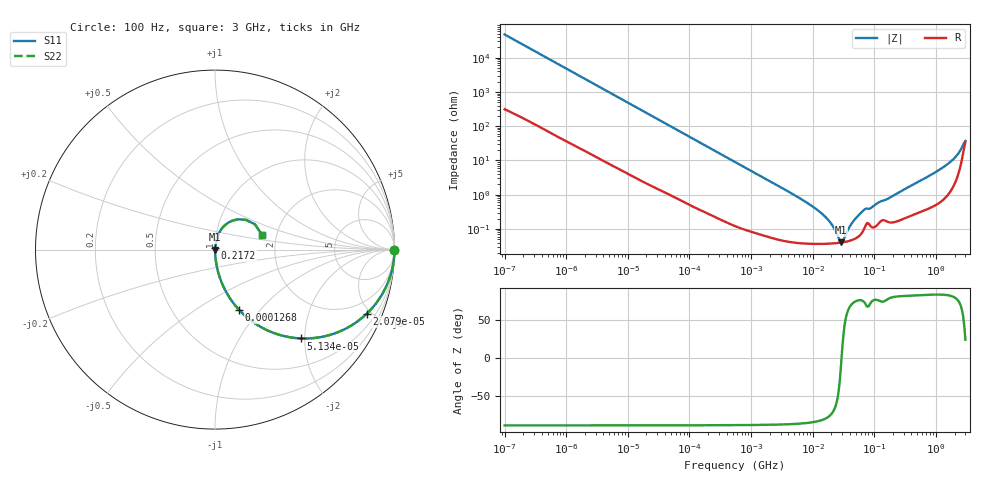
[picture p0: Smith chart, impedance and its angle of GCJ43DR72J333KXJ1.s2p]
!Murata Part Number: GCJ43DR72J333KXJ1
!These Parameters are Measured in Series Mode Connection
!Data Generated on Mar 13, 2026
!  o--ll--o
!Port1  Port2
!  o------o
!Operation Temp=25[degC], DC Bias Voltage=0[V]
!Freq. Start=100[Hz] Stop=3[GHz] 401[Steps]
# Hz S RI R 50
!Freq.(Hz) S11(Real) S11(Imag) S21(Real) S21(Imag) S12(Real) S12(Imag) S22(Real) S22(Imag)
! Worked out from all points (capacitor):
!   401 points, 100 Hz to 3 GHz, reference 50 ohm
!   read as one part in series: C = 33.4 nF near 109 Hz
!   lowest |Z| = 40.6 mohm at 28.73 MHz (marker M1)
!   series resonance near 29.37 MHz, so ESL is about 880 pH
!   S11 on the Smith chart (normalised r, x): 100 Hz: open; 20.79 kHz: 1.04, -4.70; 51.34 kHz: 1.02, -1.92; 126.8 kHz: 1.01, -0.78; 217.2 MHz: 1.00, +0.02; 3 GHz: 1.68, +0.30
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100  1 -0.0021  1.82e-05 0.0021  1.82e-05 0.0021  1 -0.0021
1788  0.9983 -0.0369  0.00166 0.0369  0.00166 0.0369  0.9983 -0.0369
6790  0.9798 -0.1367  0.0202 0.1367  0.0202 0.1367  0.9798 -0.1367
20793  0.8448 -0.3578  0.1552 0.3578  0.1552 0.3578  0.8448 -0.3578
31977  0.6999 -0.4538  0.3001 0.4538  0.3001 0.4538  0.6999 -0.4538
51340  0.4786 -0.4947  0.5214 0.4947  0.5214 0.4947  0.4786 -0.4947
126767  0.1346 -0.3361  0.8654 0.3361  0.8654 0.3361  0.1346 -0.3361
231582  0.046 -0.2039  0.954 0.2039  0.954 0.2039  0.046 -0.2039
547723  0.0094 -0.0901  0.9906 0.0901  0.9906 0.0901  0.0094 -0.0901
9794414  0.000387 -0.00459  0.9996 0.00459  0.9996 0.00459  0.000387 -0.00459
1.789277e7  0.000373 -0.00178  0.9996 0.00178  0.9996 0.00178  0.000373 -0.00178
2.12544e7  0.000378 -0.00114  0.9996 0.00114  0.9996 0.00114  0.000378 -0.00114
2.872754e7  0.000399 -7.66e-05  0.9996 7.66e-05  0.9996 7.66e-05  0.000399 -7.66e-05
3.131008e7  0.000409 0.000223  0.9996 -0.000223  0.9996 -0.000223  0.000409 0.000223
4.418008e7  0.000482 0.00148  0.9995 -0.00148  0.9995 -0.00148  0.000482 0.00148
6.508213e7  0.000858 0.00323  0.9991 -0.00323  0.9991 -0.00323  0.000858 0.00323
1.751444e8  0.00161 0.0079  0.9984 -0.0079  0.9984 -0.0079  0.00161 0.0079
2.172002e8  0.00169 0.00999  0.9983 -0.00999  0.9983 -0.00999  0.00169 0.00999
1.382454e9  0.0121 0.0659  0.9879 -0.0659  0.9879 -0.0659  0.0121 0.0659
2.219584e9  0.0496 0.1306  0.9504 -0.1306  0.9504 -0.1306  0.0496 0.1306
2.636591e9  0.1291 0.1688  0.8709 -0.1688  0.8709 -0.1688  0.1291 0.1688
3e9  0.2624 0.0828  0.7376 -0.0828  0.7376 -0.0828  0.2624 0.0828
